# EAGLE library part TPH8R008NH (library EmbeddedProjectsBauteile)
N-Channel MOSFET
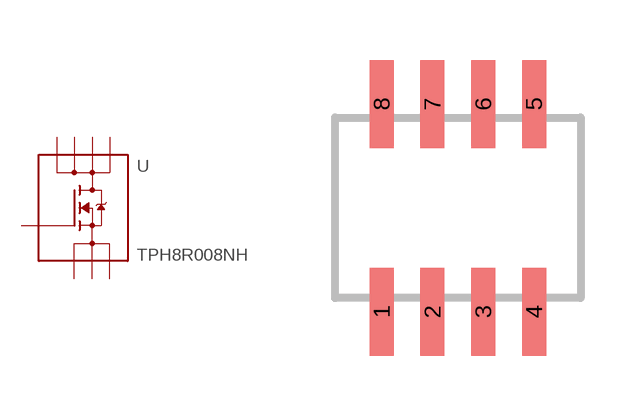
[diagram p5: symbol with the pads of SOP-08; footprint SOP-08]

Designator prefix -

## TPH8R008NH (EP: 400964)  [SOP-08]
1  S1  pas
2  S2  pas
3  S3  pas
4  G  pas
5  D1  pas
6  D2  pas
7  D3  pas
8  D4  pas

## Footprint SOP-08 (pad centres in mm)
smd 0.6 x 2.2: 1 -1.905,-2.6; 2 -0.635,-2.6; 3 0.635,-2.6; 4 1.905,-2.6; 5 1.905,2.6; 6 0.635,2.6; 7 -0.635,2.6; 8 -1.905,2.6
